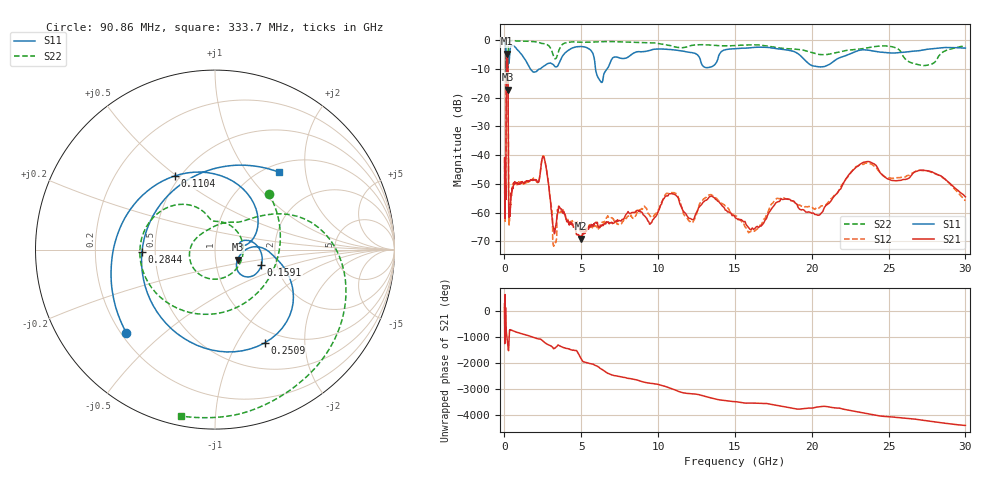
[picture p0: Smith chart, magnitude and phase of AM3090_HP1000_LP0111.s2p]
! Date/Time: Thu, Feb 28, 2019 2:02 PM
! Network Analyzer: Agilent Technologies E8364B Rev: A.07.50.67
! Sweep from 0.010 to 30.000 GHz, 1601 Points, Sweep Type: LOG
! Power Supply: 5.023 V, 0.002 A
# Hz S DB R 50
!freq MagS11 AngS11 MagS21 AngS21 MagS12 AngS12 MagS22 AngS22
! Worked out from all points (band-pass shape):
!   1601 points, 10 MHz to 30 GHz, reference 50 ohm
!   highest |S21| = -4.78 dB at 164 MHz (marker M1); lowest = -69.0 dB at 4.977 GHz (marker M2)
!   |S21| within 3 dB of the highest: 122.7 MHz to 219.7 MHz (96.94 MHz wide, 56.6 % of centre)
!   lowest |S11| = -17.2 dB at 198.3 MHz (marker M3), VSWR 1.32, Z = 63.9 - j7.26 ohm
!   |S11| at or under -10 dB: 119.3 MHz to 222.4 MHz (103.1 MHz wide, 60.3 % of centre); 1.676 GHz to 2.349 GHz (672.6 MHz wide, 33.4 % of centre); 5.925 GHz to 6.693 GHz (767.8 MHz wide, 12.2 % of centre)
!   |S22| runs from -18.8 to -0.2 dB; largest |S21 - S12| = 0.015
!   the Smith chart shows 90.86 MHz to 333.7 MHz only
!   S11 on the Smith chart (normalised r, x): 90.86 MHz: 0.22, -0.38; 110.4 MHz: 0.47, +0.49; 159.1 MHz: 1.66, -0.31; 250.9 MHz: 0.82, -1.31; 284.4 MHz: 0.42, -0.01; 333.7 MHz: 1.14, +1.43
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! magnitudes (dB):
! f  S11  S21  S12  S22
! 10 MHz  -0.3  -41.0  -40.9  -0.6
! 38.04 MHz  -0.5  -61.3  -61.2  -1.4
! 90.86 MHz  -3.4  -46.5  -48.0  -7.3
! 110.4 MHz  -6.6  -17.7  -17.7  -7.6
! 144.7 MHz  -12.8  -5.0  -5.0  -15.9
! 159.1 MHz  -11.3  -4.8  -4.8  -16.0
! 164 MHz  -11.3  -4.8  -4.8  -15.8
! 198.3 MHz  -17.2  -5.5  -5.4  -18.7
! 228.2 MHz  -8.8  -10.5  -10.5  -12.2
! 250.9 MHz  -4.6  -33.5  -33.3  -3.0
! 284.4 MHz  -7.8  -60.0  -60.1  -1.0
! 333.7 MHz  -5.1  -60.0  -60.8  -0.5
! 550.5 MHz  -2.0  -51.6  -50.4  -0.3
! 2.084 GHz  -10.9  -48.7  -49.2  -0.7
! 2.61 GHz  -9.0  -41.6  -41.3  -1.3
! 3.269 GHz  -9.1  -67.2  -70.8  -6.5
! 4.977 GHz  -2.3  -69.0  -66.1  -0.8
! 7.926 GHz  -6.3  -60.5  -62.1  -0.7
! 10.86 GHz  -3.4  -53.4  -53.0  -2.0
! 16.13 GHz  -2.7  -65.3  -66.7  -1.7
! 23.48 GHz  -3.5  -42.4  -42.8  -2.9
! 30 GHz  -2.8  -54.5  -55.8  -2.2
